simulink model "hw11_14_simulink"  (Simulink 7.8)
settings: Solver=ode45  StartTime=0.0  StopTime=50.0  RelTol=1e-3

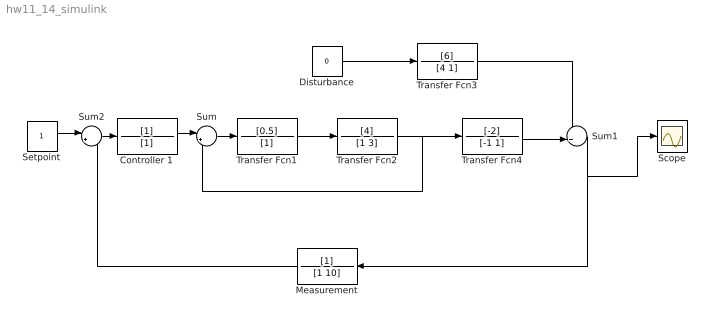
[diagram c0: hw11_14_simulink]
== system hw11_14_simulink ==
  Controller 1 : TransferFcn  Denominator=[1]
  Disturbance : Constant  Value=0
  Measurement : TransferFcn  Denominator=[1 10]
  Scope : Scope
  Setpoint : Constant
  Sum : Sum  Inputs=|+-
  Sum1 : Sum  Inputs=++|
  Sum2 : Sum  Inputs=|+-
  Transfer Fcn1 : TransferFcn  Numerator=[0.5]  Denominator=[1]
  Transfer Fcn2 : TransferFcn  Numerator=[4]  Denominator=[1 3]
  Transfer Fcn3 : TransferFcn  Numerator=[6]  Denominator=[4 1]
  Transfer Fcn4 : TransferFcn  Numerator=[-2]  Denominator=[-1 1]
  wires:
  Transfer Fcn1/1 -> Transfer Fcn2/1
  Controller 1/1 -> Sum/1
  Sum/1 -> Transfer Fcn1/1
  Transfer Fcn2/1 -> Transfer Fcn4/1, Sum/2
  Transfer Fcn4/1 -> Sum1/2
  Transfer Fcn3/1 -> Sum1/1
  Disturbance/1 -> Transfer Fcn3/1
  Sum1/1 -> Measurement/1, Scope/1
  Setpoint/1 -> Sum2/1
  Sum2/1 -> Controller 1/1
  Measurement/1 -> Sum2/2
